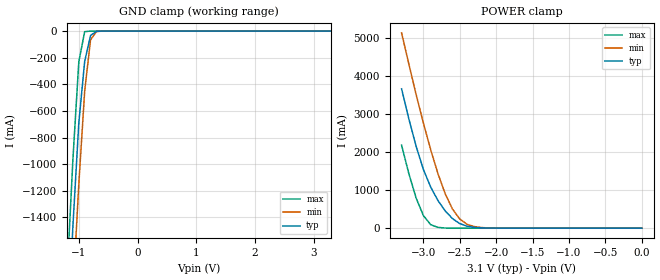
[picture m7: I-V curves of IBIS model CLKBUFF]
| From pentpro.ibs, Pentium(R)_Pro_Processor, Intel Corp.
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[Model]   CLKBUFF
Model_type   Input
Vinl = 0.8v
Vinh = 2.0v
|variable   typ   min   max
C_comp   2.1p  1.9p  2.3p
|variable   typ   min   max
[Voltage Range]   3.1v  2.845 3.255
|Variable   typ   min   max
[Temperature Range] 80   0   100
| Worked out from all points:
|   GND clamp passes 1 mA (typ) near -0.65 V on its own axis
|   POWER clamp passes 1 mA (typ) near -1.98 V on its own axis
[GND_Clamp]
|Voltage  I(typ)   I(min)   I(max)
-2V       -9.98A     -10.4A     -9.53A
-1.2V     -2.35A     -2.86A     -1.84A
-1.1V     -1.46A     -1.97A     -960mA
-1V       -690mA     -1.15A     -230mA
-900mV    -227mA     -450mA     -4.26mA
-800mV    -32.9mA    -65.7mA    -74.4uA
-700mV    -1.81mA    -3.61mA    -7.46uA
3.3V      0A         0A         0A
[POWER_Clamp]
|Voltage  I(typ)   I(min)   I(max)
-3.3V     3.66A      5.13A      2.18A
-3.2V     2.87A      4.31A      1.43A
-3.1V     2.15A      3.51A      790mA
-3V       1.54A      2.76A      330mA
-2.9V     1.08A      2.06A      91.7mA
-2.8V     725mA      1.43A      19.7mA
-2.7V     452mA      900mA      3.84mA
-2.6V     250mA      500mA      740uA
-2.5V     120mA      240mA      140uA
-2.3V     20.5mA     41mA       0A
-2.1V     2.97mA     5.94mA     0A
0V        0A         0A         0A
